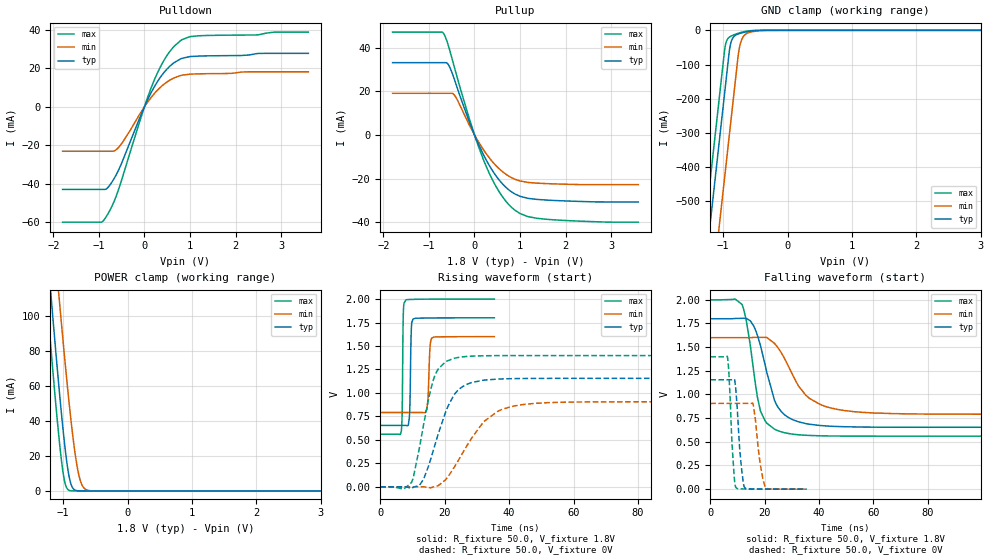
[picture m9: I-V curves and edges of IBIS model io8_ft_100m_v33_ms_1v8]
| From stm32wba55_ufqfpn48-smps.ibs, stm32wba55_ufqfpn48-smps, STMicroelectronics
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[Model]   io8_ft_100m_v33_ms_1v8
Model_type I/O
Polarity   Non-Inverting
Enable   Active-Low
| CAP_THRESHOLD on pad IOFT is "UDTCAPC" :
| Rising=30.0% of vddiom   Falling=70.0% of vddiom
| C_comp min and max val. don't necessarily correlate with the min and max pvt
| but are the smallest and greatest pad capacitance found.
| var   typ   min   max
C_comp   2.30360pF  2.19151pF  2.50009pF
|C_comp_pullup   1.45390pF  1.38820pF  1.55640pF
|C_comp_pulldown   849.70020fF  803.31002fF  943.68706fF
Vinl = 800.0mV
Vinh = 1.0V
Vmeas = 900.0mV   | Reference voltage for timing measurements
Cref  = 50.0pF   | Timing specification test load capacitance value
Rref  = 1.0MOhm   | Timing specification test load resistance value
Vref  = 990.0mV   | Timing specification test load voltage
[Model Spec]
| TIME_THRESHOLD on pin ZIV33M is "CMOS" :
| Rising=50.0% of vddiom   Falling=50.0% of vddiom
Vinl 697.50000mV 636.50000mV 765.50000mV
Vinh 1.08850V 942.50000mV 1.21750V
| variable   typ   min   max
[Temperature Range] 25.0 140.0 -40.0
| variable   typ   min   max
[Voltage Range] 1.8V 1.6V 2.0V
| variable   typ   min   max
[POWER Clamp Reference] 1.8V 1.6V 2.0V
| variable   typ   min   max
[GND Clamp Reference] 0V 0V 0V
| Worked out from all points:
|   slope of the pulldown table from 0 to 0.27 V, typ, clamps not added: 21.7 ohm
|   slope of the pullup table from 0 to 0.27 V, typ, clamps not added: 22.5 ohm
|   GND clamp passes 1 mA (typ) near -0.51 V on its own axis
|   POWER clamp passes 1 mA (typ) near -0.83 V on its own axis
|   rising waveform, R_fixture 50.0, V_fixture 1.8V: 20-80 % time 334ps typ, 527ps min, 257ps max; typ from 0.654 V to 1.8 V
|   falling waveform, R_fixture 50.0, V_fixture 1.8V: 20-80 % time 6.65ns typ, 10.6ns min, 4.64ns max; typ from 1.8 V to 0.654 V
|   rising waveform, R_fixture 50.0, V_fixture 0V: 20-80 % time 6.96ns typ, 10.9ns min, 4.96ns max; typ from 0 V to 1.16 V
|   falling waveform, R_fixture 50.0, V_fixture 0V: 20-80 % time 1.72ns typ, 2.26ns min, 1.41ns max; typ from 1.16 V to 0 V
[POWER Clamp]
-1.8V     396.4mA    438.1mA    365.5mA
-1.26V    143.5mA    194.6mA    112.6mA
-1.19V    112.3mA    164.2mA    81.56mA
-1.06V    57.23mA    109.3mA    28.68mA
-1.02V    41.75mA    93.06mA    15.5mA
-980mV    27.6mA     77.28mA    5.935mA
-910mV    8.693mA    51.24mA    382.3uA
-850mV    1.642mA    31.41mA    23.97uA
-760mV    69.41uA    9.714mA    358.6nA
-700mV    7.83uA     2.919mA    21.79nA
-620mV    424.6nA    410.3uA    573.9pA
3.6V      0A         0A         0A
[GND Clamp]
-1.8V     -1.583A    -1.83A     -1.456A
-1.43V    -953.9mA   -1.201A    -826.8mA
-1.24V    -630.9mA   -877.8mA   -503.8mA
-1.05V    -307.9mA   -554.8mA   -180.8mA
-970mV    -171.9mA   -418.8mA   -48.31mA
-910mV    -69.87mA   -316.8mA   -20.91mA
-880mV    -36.5mA    -265.8mA   -17.19mA
-830mV    -17.68mA   -180.8mA   -12.97mA
-750mV    -9.66mA    -53.66mA   -7.697mA
-690mV    -6.479mA   -19.19mA   -4.622mA
-600mV    -3.058mA   -6.478mA   -1.59mA
3.6V      1.279nA    1.39uA     517.2pA
| variable   typ   min   max
[Pullup Reference] 1.8V 1.6V 2.0V
| variable   typ   min   max
[Pulldown Reference] 0V 0V 0V
[Pullup]
-1.8V     33.11mA    19.07mA    47.12mA
-680mV    33.11mA    19.07mA    46.55mA
-570mV    32.06mA    19.07mA    40.63mA
-430mV    24.73mA    17.91mA    30.12mA
-120mV    6.338mA    4.782mA    7.854mA
200mV     -9.203mA   -6.891mA   -11.54mA
530mV     -20.35mA   -15.28mA   -25.66mA
690mV     -24.02mA   -18.04mA   -30.41mA
880mV     -26.99mA   -20.26mA   -34.39mA
1.18V     -29.09mA   -21.8mA    -37.49mA
1.56V     -29.85mA   -22.32mA   -38.64mA
3.6V      -30.74mA   -22.8mA    -40.02mA
[Pulldown]
-1.8V     -42.97mA   -23.15mA   -59.99mA
-950mV    -42.97mA   -23.15mA   -59.99mA
-850mV    -42.87mA   -23.15mA   -57.45mA
-670mV    -37.41mA   -23.03mA   -49.3mA
-550mV    -31.91mA   -20.61mA   -41.6mA
10mV      539.8uA    356.7uA    722uA
230mV     10.88mA    7.174mA    14.64mA
500mV     19.69mA    12.93mA    26.79mA
790mV     24.78mA    16.15mA    34.26mA
1V        26.02mA    16.89mA    36.38mA
1.18V     26.27mA    17.05mA    36.82mA
3.6V      27.7mA     18.13mA    38.74mA
[Ramp]
dV/dt_r 693.10568mV/6.84545ns 543.2516mV/10.6111ns 838.8428mV/4.87351ns
dV/dt_f 687.69012mV/6.60504ns 484.94283mV/10.54982ns 864.0014mV/4.5372ns
R_load = 50.0
| Removed startup time: 0s 0s 0s  .
| Removed end time: 35.4ns.
[Rising Waveform]
R_fixture   = 50.0
V_fixture   = 1.8V
V_fixture_min = 1.6V
V_fixture_max = 2.0V
0s        653.8mV    791.8mV    560mV
6.5ns     653.8mV    791.8mV    585.7mV
7.15ns    653.9mV    791.8mV    1.844V
7.95ns    653.7mV    791.8mV    1.992V
9.05ns    751.8mV    791.8mV    1.996V
9.6ns     1.646V     791.8mV    1.996V
10.15ns   1.787V     791.8mV    1.996V
14.45ns   1.798V     824.5mV    1.999V
15.9ns    1.798V     1.584V     1.999V
35.4ns    1.8V       1.6V       2V
| Removed startup time: 0s 0s 0s  .
| Removed end time: 198.4ns.
[Falling Waveform]
R_fixture   = 50.0
V_fixture   = 1.8V
V_fixture_min = 1.6V
V_fixture_max = 2.0V
0s        1.8V       1.6V       2V
11.65ns   1.804V     1.6V       1.952V
14.7ns    1.779V     1.6V       1.522V
17.3ns    1.628V     1.603V     976.8mV
18.45ns   1.517V     1.603V     824.3mV
23.6ns    940.1mV    1.54V      634mV
27.4ns    784.1mV    1.375V     595.1mV
36.45ns   685.9mV    959.2mV    567.5mV
49.7ns    659.3mV    828.3mV    560.8mV
198.4ns   653.8mV    791.8mV    560mV
| Removed startup time: 0s 0s 0s  .
| Removed end time: 198.35ns.
[Rising Waveform]
R_fixture   = 50.0
V_fixture   = 0V
V_fixture_min = 0V
V_fixture_max = 0V
0s        4.767nV    680.3nV    4.105nV
7.15ns    1.579uV    679.1nV    -25.22mV
9.7ns     -18.94mV   684.2nV    46.41mV
13.45ns   81.42mV    155.1uV    664.6mV
16.8ns    427mV      346.5uV    1.172V
20.25ns   793.4mV    74.14mV    1.331V
23.45ns   1.003V     236.3mV    1.373V
32.4ns    1.137V     701.7mV    1.396V
45.7ns    1.154V     882.3mV    1.398V
198.3ns   1.155V     905.4mV    1.398V
| Removed startup time: 0s 0s 0s  .
| Removed end time: 35.4ns.
[Falling Waveform]
R_fixture   = 50.0
V_fixture   = 0V
V_fixture_min = 0V
V_fixture_max = 0V
0s        1.155V     905.5mV    1.398V
6.3ns     1.155V     905.5mV    1.398V
8ns       1.155V     905.5mV    478.4mV
9.4ns     1.051V     905.5mV    18.05mV
10.85ns   413.1mV    905.5mV    3.407mV
12.55ns   20.57mV    905.5mV    1.867mV
15.65ns   1.772mV    906.4mV    659.4uV
18.6ns    764.8uV    227.6mV    380.2uV
20.45ns   547.8uV    16.81mV    278.1uV
35.4ns    79.53uV    342.3uV    22.68uV
